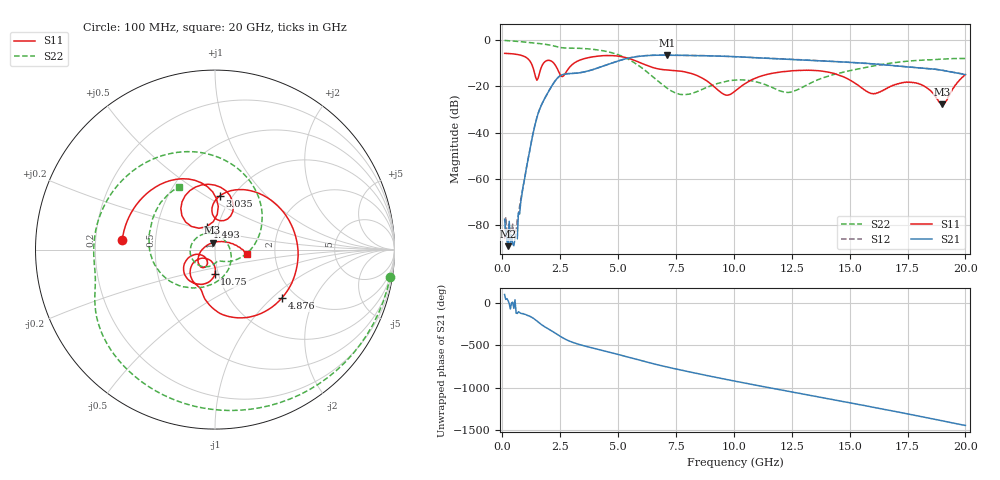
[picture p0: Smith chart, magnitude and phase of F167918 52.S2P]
!  2-Port S-parameters saved by WinCal
! VAR MeasName=S-Parameters (CALIBRATED_DATA) read from VNA (N5242A)
! VAR MeasDate=2016-11-22 10:27:20
! VAR NAME=F167918 52
! VAR FILENAME=F167918 52.S2P
! VAR DATE=2016-11-22 10:27:21
! VAR PHYS_PORTS=1,2
# Hz S DB R 50
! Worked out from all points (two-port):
!   401 points, 100 MHz to 20 GHz, reference 50 ohm
!   highest |S21| = -6.46 dB at 7.115 GHz (marker M1); lowest = -89.1 dB at 249.2 MHz (marker M2)
!   |S21| within 3 dB of the highest: 4.848 GHz to 14.79 GHz (9.944 GHz wide, 101 % of centre)
!   lowest |S11| = -27.8 dB at 19 GHz (marker M3), VSWR 1.09, Z = 48.5 + j3.74 ohm
!   |S11| at or under -10 dB: 1.252 GHz to 1.778 GHz (525.7 MHz wide, 34.7 % of centre); 2.229 GHz to 3.087 GHz (857.9 MHz wide, 32.3 % of centre); 6.021 GHz to end of sweep
!   |S22| runs from -23.5 to -0.1 dB; largest |S21 - S12| = 0.0038
!   S11 on the Smith chart (normalised r, x): 100 MHz: 0.32, +0.05; 1.493 GHz: 0.88, +0.23; 3.035 GHz: 0.88, +0.58; 4.876 GHz: 1.69, -1.16; 10.75 GHz: 0.96, -0.27; 20 GHz: 1.43, -0.08
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1e8  -5.68 174.1  -77.44 99.9  -86.01 113.6  -0.10 -8.7
2.4925e8  -5.74 165.2  -89.06 29.2  -84.62 22.9  -0.19 -21.0
6.4725e8  -6.16 140.5  -85.89 -123.6  -77.14 -89.5  -0.48 -52.4
1.493e9  -17.31 109.5  -33.49 147.4  -33.50 147.5  -1.33 -110.2
2.289e9  -10.80 70.4  -17.51 3.6  -17.51 3.6  -2.63 -154.8
2.5875e9  -15.73 80.1  -14.94 -48.1  -14.93 -48.0  -3.27 -166.3
3.03525e9  -10.40 84.6  -14.37 -105.0  -14.36 -105.1  -3.41 176.9
3.43325e9  -8.30 58.2  -13.92 -139.1  -13.92 -139.1  -3.55 159.5
4.876e9  -6.75 -36.0  -9.36 120.4  -9.36 120.5  -5.84 86.6
5.72175e9  -8.74 -83.0  -7.20 58.4  -7.18 58.5  -9.86 35.1
6.7665e9  -12.47 -108.8  -6.47 -14.7  -6.45 -14.7  -18.02 -28.2
7.11475e9  -12.87 -113.3  -6.46 -36.9  -6.45 -36.9  -20.77 -46.4
8.30875e9  -14.87 -140.0  -6.63 -107.8  -6.60 -107.7  -22.58 -88.1
1.005e10  -22.02 -96.5  -7.11 155.6  -7.12 155.7  -17.26 -159.1
1.07465e10  -17.24 -90.7  -7.48 118.7  -7.44 118.8  -17.51 166.1
1.23385e10  -13.40 -115.9  -8.23 36.7  -8.18 36.6  -22.59 41.2
1.338325e10  -13.06 -134.9  -8.72 -16.7  -8.68 -16.8  -18.19 -48.2
1.49255e10  -16.74 -163.9  -9.54 -95.5  -9.51 -95.9  -13.31 -106.0
1.67165e10  -20.31 -117.6  -10.80 170.4  -10.84 170.5  -10.00 -149.7
1.796025e10  -18.70 -144.5  -12.00 105.1  -11.91 105.2  -8.70 177.9
1.9005e10  -27.79 109.5  -13.01 46.6  -12.98 46.5  -8.17 150.3
2e10  -14.88 -8.2  -14.84 -8.1  -14.77 -7.9  -7.89 120.0
